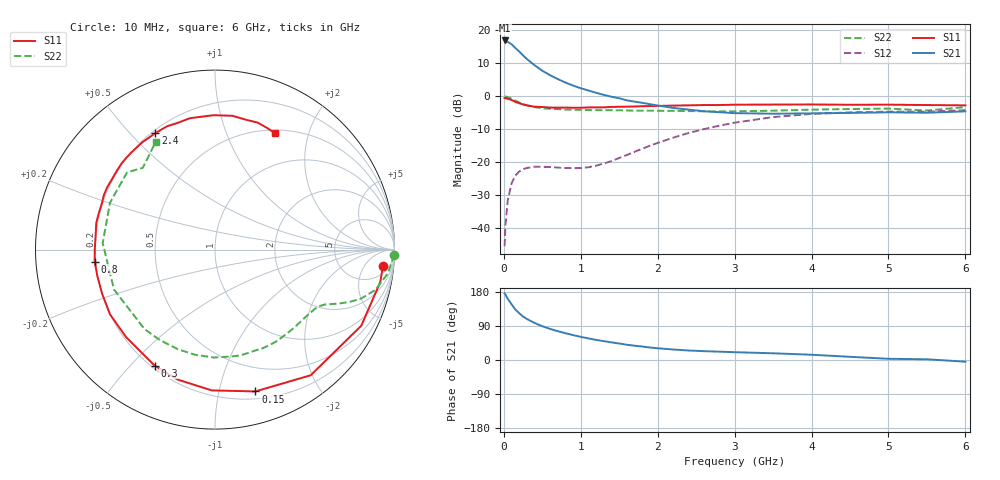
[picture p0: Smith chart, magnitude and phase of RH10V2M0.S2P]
! SIEMENS Small Signal Semiconductors
! BFR106
! Si NPN RF Bipolar Junction Transistor in SOT23
! VCE = 10 V  IC = 2 mA
! Common Emitter S-Parameters:  August  1996
# GHz  S  MA  R  50
!  f  S11  S21  S12  S22
! GHz  MAG  ANG  MAG  ANG  MAG  ANG  MAG  ANG
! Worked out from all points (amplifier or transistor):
!   36 points, 10 MHz to 6 GHz, reference 50 ohm
!   highest |S21| = 17.0 dB at 10 MHz (marker M1)
!   |S21| within 3 dB of that: start of sweep to 183.2 MHz
!   unconditionally stable (mu >= 1): 786.2 MHz to 1.802 GHz; 4.205 GHz to end of sweep
!   at 250 MHz: K = 0.32, MSG = 17.3 dB, |S12| = -22.1 dB
!   at 1.4 GHz: K = 1.23, MAG = 6.9 dB, |S12| = -19.7 dB
!   at 6 GHz: K = 1.02, MAG = -1.0 dB, |S12| = -4.2 dB
!   S11 on the Smith chart (normalised r, x): 10 MHz: 9, -15; 150 MHz: 0.27, -1.29; 300 MHz: 0.21, -0.59; 800 MHz: 0.20, -0.05; 2.4 GHz: 0.21, +0.59; 6 GHz: 0.54, +1.50
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0.01  0.9401 -5.6  7.049 175.7  0.0053 87.5  0.997 -1.6
0.02  0.9385 -11.1  6.969 172.9  0.0107 84.5  0.9909 -3.2
0.05  0.9187 -27.5  6.733 161.9  0.026 75.0  0.9734 -7.7
0.1  0.8801 -52.7  6.173 147.1  0.0477 62.6  0.9215 -14.1
0.15  0.8216 -74.1  5.412 133.2  0.0626 51.9  0.8581 -18.6
0.2  0.7847 -91.3  4.789 123.5  0.0721 44.7  0.8053 -21.2
0.25  0.7534 -106.1  4.186 114.6  0.0783 38.9  0.7604 -23.2
0.3  0.7286 -117.5  3.676 108.2  0.0816 35.4  0.7293 -24.5
0.4  0.695 -135.5  2.962 97.8  0.0852 30.3  0.6851 -26.5
0.5  0.6874 -148.3  2.447 89.1  0.0851 28.3  0.6598 -28.6
0.6  0.6751 -158.6  2.096 82.1  0.0844 28.4  0.6462 -30.9
0.8  0.6739 -174.3  1.618 70.7  0.0815 32.9  0.6297 -36.3
1.1  0.678 167.4  1.224 57.0  0.0837 48.5  0.6183 -45.8
1.6  0.6953 145.5  0.869 40.2  0.1286 71.0  0.6104 -64.3
2.2  0.7223 124.1  0.666 27.7  0.2353 72.7  0.6014 -90.4
2.4  0.7289 117.2  0.628 25.1  0.2767 69.9  0.5964 -100.7
3  0.7453 100.8  0.555 20.6  0.3977 57.2  0.5919 -131.6
3.5  0.7489 90.6  0.544 17.7  0.4836 44.9  0.605 -158.4
4.5  0.7437 76.6  0.56 8.4  0.5701 21.7  0.6407 155.9
5  0.7465 71.4  0.571 3.2  0.5853 12.6  0.652 138.7
5.5  0.7364 66.3  0.563 1.9  0.584 8.1  0.6078 131.5
6  0.7291 62.9  0.591 -4.5  0.6162 -0.2  0.6855 118.8
